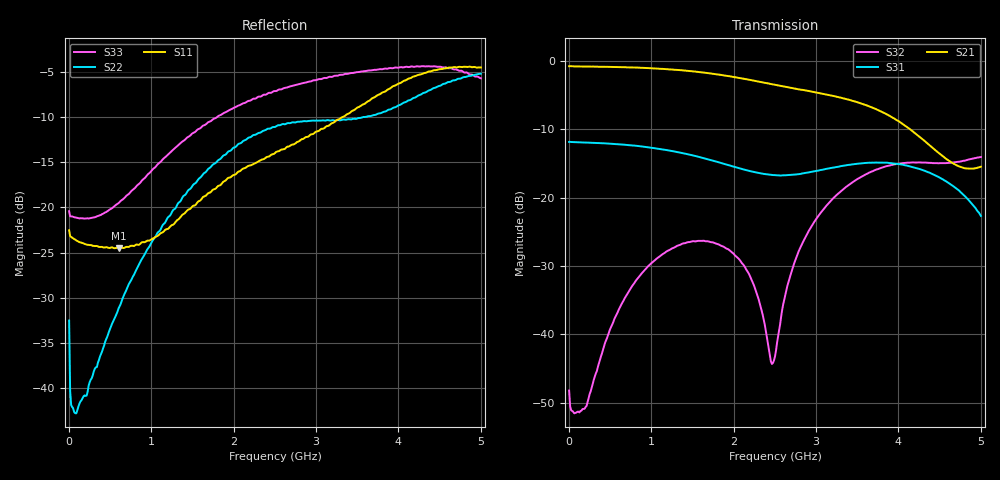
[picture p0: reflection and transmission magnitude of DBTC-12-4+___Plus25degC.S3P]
! Mini-Circuits
! S3P DATA File Format
! Type: Directional Coupler
! Model:DBTC-12-4+
! PINOUT: IN PORT=PORT1 , OUT PORT=PORT2 , COUPLED PORT=PORT3
! TEST CONDITIONS: INPUT POWER = 0 dBm @ Temperature = + 25 deg C
! 401 Frequency points
! All S Parameters are in dB deg format
# MHz S DB R 50
!FREQ	MAG(S11)PHS(S11)MAG(S12)PHS(S12)MAG(S13)PHS(S13)
!	MAG(S21)PHS(S21)MAG(S22)PHS(S22)MAG(S23)PHS(S23)
!	MAG(S31)PHS(S31)MAG(S32)PHS(S32)MAG(S33)PHS(S33)
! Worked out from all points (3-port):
!   401 points, 5 MHz to 5 GHz, reference 50 ohm
!   strongest paths, dB at 5 MHz, 1.254 GHz, 2.502 GHz, 3.751 GHz, 5 GHz:
!     S21: -0.8, -1.2, -3.5, -7.2, -15.4
!     S31: -11.8, -13.2, -16.7, -14.9, -22.7
!     S32: -48.2, -27.4, -43.2, -15.8, -14.0
!   lowest |S11| = -24.5 dB at 604.4 MHz (marker M1), VSWR 1.13, Z = 48 + j5.47 ohm
!   |S11| at or under -10 dB: start of sweep to 3.324 GHz
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5  -22.53 164.6  -0.73 0.7  -11.84 -180.0
   -0.75 0.6  -32.52 110.7  -48.51 45.4
   -11.83 180.0  -48.23 43.9  -20.42 165.2
92.41  -23.66 164.1  -0.76 -8.8  -11.89 -192.8
       -0.78 -8.8  -42.79 100.0  -52.96 -52.0
       -11.88 167.1  -51.45 -49.5  -21.12 171.3
604.4  -24.53 106.8  -0.86 -57.1  -12.18 -262.4
       -0.88 -57.0  -31.19 -52.8  -36.57 -240.4
       -12.17 97.5  -36.45 -241.3  -19.53 142.6
1628.38  -18.85 23.2  -1.65 -155.7  -14.20 -392.4
         -1.67 -155.5  -16.32 -201.6  -26.26 -399.4
         -14.18 -32.2  -26.29 -399.2  -10.96 33.8
2140.36  -15.64 -33.4  -2.59 -205.1  -15.94 -445.8
         -2.62 -204.8  -12.56 -265.3  -30.19 -466.7
         -15.91 -85.6  -30.21 -466.5  -8.42 -32.8
2502.5  -13.99 -77.2  -3.42 -239.1  -16.69 -476.4
        -3.46 -238.8  -11.10 -309.9  -43.55 -407.2
        -16.69 -116.4  -43.23 -410.9  -7.12 -78.6
2814.69  -12.52 -113.2  -4.14 -267.8  -16.46 -501.9
         -4.19 -267.6  -10.50 -347.6  -27.20 -398.9
         -16.51 -142.1  -27.18 -399.9  -6.31 -117.2
3489.01  -9.03 -186.4  -5.96 -333.0  -15.04 -571.2
         -5.97 -333.0  -10.20 -427.1  -17.36 -485.8
         -15.04 -211.2  -17.36 -485.7  -5.04 -194.4
4325.68  -5.12 -277.4  -11.72 -411.0  -16.08 -682.0
         -11.78 -411.0  -7.28 -532.8  -14.93 -589.5
         -16.09 -321.5  -14.85 -589.5  -4.40 -280.6
5000  -4.51 -347.6  -15.30 -426.4  -22.70 -799.7
      -15.45 -425.9  -5.20 -619.6  -14.13 -655.6
      -22.66 -438.8  -14.04 -655.9  -5.71 -339.8
